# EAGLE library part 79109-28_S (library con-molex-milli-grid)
RECEPTACAL
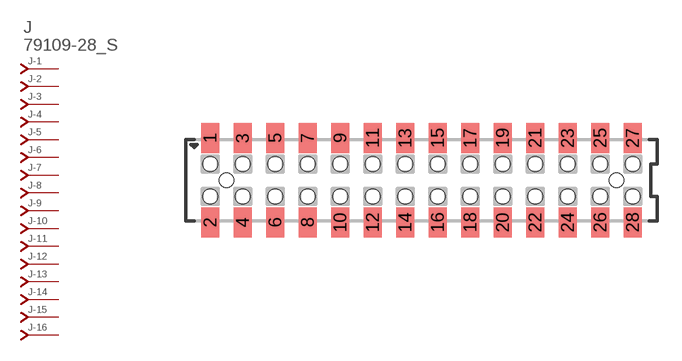
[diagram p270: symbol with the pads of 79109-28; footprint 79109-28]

Designator prefix J; gates -1=J-NV -2=J-N -3=J-N -4=J-N -5=J-N -6=J-N -7=J-N -8=J-N -9=J-N -10=J-N -11=J-N -12=J-N -13=J-N -14=J-N -15=J-N -16=J-N -17=J-N -18=J-N -19=J-N -20=J-N -21=J-N -22=J-N -23=J-N -24=J-N -25=J-N -26=J-N -27=J-N -28=J-N

## 79109-28_S  [79109-28]
1  -1:J  pas
2  -2:J  pas
3  -3:J  pas
4  -4:J  pas
5  -5:J  pas
6  -6:J  pas
7  -7:J  pas
8  -8:J  pas
9  -9:J  pas
10  -10:J  pas
11  -11:J  pas
12  -12:J  pas
13  -13:J  pas
14  -14:J  pas
15  -15:J  pas
16  -16:J  pas
17  -17:J  pas
18  -18:J  pas
19  -19:J  pas
20  -20:J  pas
21  -21:J  pas
22  -22:J  pas
23  -23:J  pas
24  -24:J  pas
25  -25:J  pas
26  -26:J  pas
27  -27:J  pas
28  -28:J  pas

## Footprint 79109-28 (pad centres in mm)
RECEPTACAL SMD Dual Row, Vertical, Pass-Thru
smd 1.12 x 1.83: 1 -13,2.6; 2 -13,-2.6; 3 -11,2.6; 4 -11,-2.6; 5 -9,2.6; 6 -9,-2.6; 7 -7,2.6; 8 -7,-2.6; 9 -5,2.6; 10 -5,-2.6; 11 -3,2.6; 12 -3,-2.6; 13 -1,2.6; 14 -1,-2.6; 15 1,2.6; 16 1,-2.6; 17 3,2.6; 18 3,-2.6; 19 5,2.6; 20 5,-2.6; 21 7,2.6; 22 7,-2.6; 23 9,2.6; 24 9,-2.6; 25 11,2.6; 26 11,-2.6; 27 13,2.6; 28 13,-2.6
hole 0.914 at -12,0
hole 0.914 at -13,1
hole 0.914 at -13,-1
hole 0.914 at -11,-1
hole 0.914 at -11,1
hole 0.914 at -9,-1
hole 0.914 at -9,1
hole 0.914 at 12,0
hole 0.914 at -7,1
hole 0.914 at -7,-1
hole 0.914 at -5,1
hole 0.914 at -5,-1
hole 0.914 at -3,1
hole 0.914 at -3,-1
hole 0.914 at -1,1
hole 0.914 at -1,-1
hole 0.914 at 1,-1
hole 0.914 at 1,1
hole 0.914 at 3,1
hole 0.914 at 3,-1
hole 0.914 at 5,1
hole 0.914 at 5,-1
hole 0.914 at 7,1
hole 0.914 at 7,-1
hole 0.914 at 9,-1
hole 0.914 at 9,1
hole 0.914 at 11,1
hole 0.914 at 13,1
hole 0.914 at 11,-1
hole 0.914 at 13,-1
